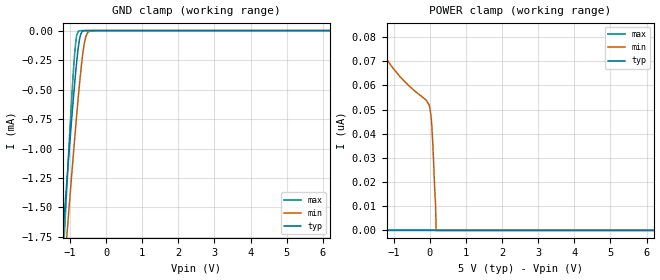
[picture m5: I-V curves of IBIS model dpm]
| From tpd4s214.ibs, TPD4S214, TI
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|   dpm Model
[Model]   dpm
Model_type   Input
Vinl = 0.4
Vinh = 1.2
|   typ   min   max
|   (nom PVT)   (fast PVT)   (slow PVT)
C_comp   3.719e-13   1.954e-13   3.837e-13
| Where nom  PVT is Nominal Process, 5V, 27C
|   Fast PVT is Strong Process,  5.5V, -40C
|   Slow PVT is Weak Process,   4.5V, 125C
[Voltage Range]   5   4.5   5.5
|Junction Temperature
[Temperature Range]   27   125   -40
[Power Clamp Reference]   5   4.5   5.5
[GND Clamp Reference]   0   0   0
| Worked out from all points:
|   GND clamp passes 1 mA (typ) near -1.02 V on its own axis
[GND Clamp]
|   Voltage   I(typ)   I(min)   I(max)
-5V       -18.24mA   -18.1mA    -26.08mA
-1.249V   -1.941mA   -2.385mA   -2.289mA
-1.139V   -1.488mA   -1.947mA   -1.628mA
-1.081V   -1.25mA    -1.716mA   -1.285mA
-941mV    -703.7uA   -1.178mA   -512.9uA
-875mV    -462.8uA   -932.7uA   -210.5uA
-819.5mV  -278.9uA   -733uA     -50.38uA
-740mV    -79.73uA   -464.2uA   -1.872uA
-644mV    -4.704uA   -191.6uA   -20.38nA
-563mV    -276.5nA   -51.3uA    0A
-396.5mV  0A         -838.1nA   0A
10V       0A         0A         0A
[POWER Clamp]
|   Voltage   I(typ)   I(min)   I(max)
-5V       12.25nA    630.7nA    0A
-4.643V   10.08nA    501.8nA    0A
-4.46V    0A         445.5nA    0A
-1.603V   0A         81.79nA    0A
-1.036V   0A         67.42nA    0A
-22.5mV   0A         51.98nA    0A
26.5mV    0A         48.08nA    0A
62.5mV    0A         41.32nA    0A
139mV     0A         15.85nA    0A
157mV     0A         10.87nA    0A
175mV     0A         0A         0A
10V       0A         0A         0A
